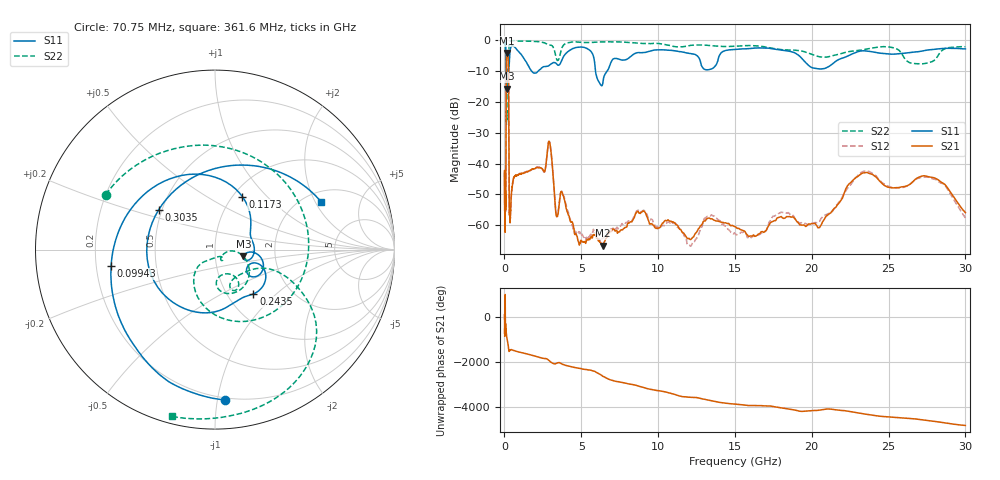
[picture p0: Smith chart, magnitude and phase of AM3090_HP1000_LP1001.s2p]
! Date/Time: Thu, Feb 28, 2019 2:02 PM
! Network Analyzer: Agilent Technologies E8364B Rev: A.07.50.67
! Sweep from 0.010 to 30.000 GHz, 1601 Points, Sweep Type: LOG
! Power Supply: 5.023 V, 0.002 A
# Hz S DB R 50
!freq MagS11 AngS11 MagS21 AngS21 MagS12 AngS12 MagS22 AngS22
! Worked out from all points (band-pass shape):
!   1601 points, 10 MHz to 30 GHz, reference 50 ohm
!   highest |S21| = -4.14 dB at 165.6 MHz (marker M1); lowest = -66.6 dB at 6.424 GHz (marker M2)
!   |S21| within 3 dB of the highest: 122.5 MHz to 252.6 MHz (130.1 MHz wide, 69.4 % of centre)
!   lowest |S11| = -15.8 dB at 153.7 MHz (marker M3), VSWR 1.39, Z = 68.5 - j5.28 ohm
!   |S11| at or under -10 dB: 118 MHz to 229.4 MHz (111.3 MHz wide, 64.1 % of centre); 1.762 GHz to 2.201 GHz (439.2 MHz wide, 22.2 % of centre); 5.925 GHz to 6.693 GHz (767.9 MHz wide, 12.2 % of centre)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
!   |S22| runs from -27.4 to -0.1 dB; largest |S21 - S12| = 0.012
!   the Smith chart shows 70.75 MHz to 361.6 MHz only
!   S11 on the Smith chart (normalised r, x): 70.75 MHz: 0.19, -1.05; 99.43 MHz: 0.26, -0.07; 117.3 MHz: 1.11, +0.73; 243.5 MHz: 1.31, -0.73; 303.5 MHz: 0.48, +0.25; 361.6 MHz: 2.46, +2.24
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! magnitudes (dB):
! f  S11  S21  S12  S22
! 10 MHz  -0.2  -43.2  -42.9  -0.6
! 38.04 MHz  -0.5  -60.1  -60.0  -1.6
! 70.75 MHz  -1.5  -52.9  -55.6  -3.3
! 86.43 MHz  -2.8  -53.3  -51.9  -4.9
! 99.43 MHz  -4.6  -33.6  -33.8  -5.6
! 117.3 MHz  -9.6  -10.2  -10.2  -12.5
! 144.7 MHz  -14.4  -4.4  -4.4  -25.7
! 153.7 MHz  -15.8  -4.2  -4.2  -21.8
! 165.6 MHz  -13.3  -4.1  -4.1  -14.5
! 243.5 MHz  -9.7  -6.1  -6.1  -12.6
! 269.1 MHz  -9.5  -12.6  -12.6  -10.0
! 303.5 MHz  -8.3  -50.5  -51.5  -1.2
! 361.6 MHz  -3.8  -58.4  -57.5  -0.4
! 550.5 MHz  -1.9  -45.7  -45.9  -0.2
! 2.084 GHz  -10.6  -41.3  -41.4  -0.5
! 2.928 GHz  -8.1  -33.0  -32.9  -1.6
! 3.402 GHz  -7.8  -57.3  -56.3  -6.3
! 6.424 GHz  -13.2  -66.6  -64.0  -0.6
! 7.926 GHz  -6.3  -60.6  -59.1  -0.7
! 16.37 GHz  -2.6  -63.5  -63.3  -1.9
! 23.59 GHz  -3.6  -42.9  -42.5  -2.9
! 30 GHz  -2.9  -55.9  -57.6  -2.2
